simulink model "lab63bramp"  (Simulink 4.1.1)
settings: Solver=ode45  StartTime=0.0  StopTime=10.0  MaxStep=.01  RelTol=1e-6
libraries: simulink3 x1

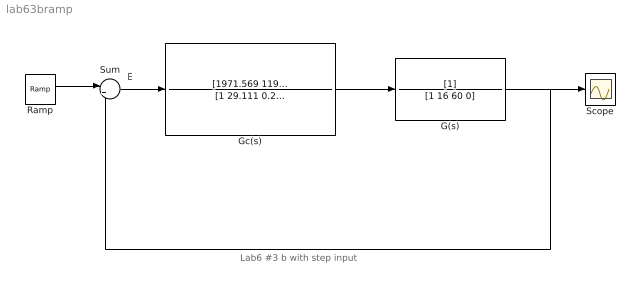
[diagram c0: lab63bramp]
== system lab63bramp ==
  note: E
  note: Lab6 #3 b with step input
  G(s) : TransferFcn  Numerator=[1]  Denominator=[1 16 60 0]  AbsoluteTolerance=auto  Realization=auto
  Gc(s) : TransferFcn  Numerator=[1971.569 11922.3 557.52]  Denominator=[1 29.111 0.29101]  AbsoluteTolerance=auto  Realization=auto
  Ramp : simulink3/Sources/Ramp  slope=1  start=0  X0=0
  Scope : Scope
  Sum : Sum  Inputs=|+-  SaturateOnIntegerOverflow=on
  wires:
  G(s)/1 -> Scope/1, Sum/2
  Gc(s)/1 -> G(s)/1
  Sum/1 -> Gc(s)/1
  Ramp/1 -> Sum/1
